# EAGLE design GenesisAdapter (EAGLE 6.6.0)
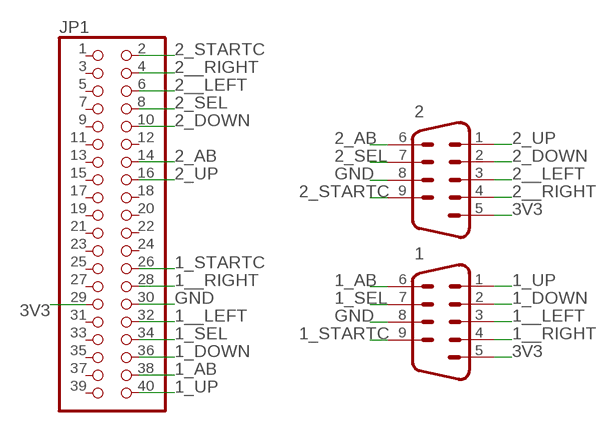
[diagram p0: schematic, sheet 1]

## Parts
1  M09H  [M09H]
2  M09H  [M09H]
JP1  PINHD-2X20  [2X20]

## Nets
1__LEFT: 1.3 JP1.32
1__RIGHT: 1.4 JP1.28
1_AB: 1.6 JP1.38
1_DOWN: 1.2 JP1.36
1_SEL: 1.7 JP1.34
1_STARTC: 1.9 JP1.26
1_UP: 1.1 JP1.40
2__LEFT: 2.3 JP1.6
2__RIGHT: 2.4 JP1.4
2_AB: 2.6 JP1.14
2_DOWN: 2.2 JP1.10
2_SEL: 2.7 JP1.8
2_STARTC: 2.9 JP1.2
2_UP: 2.1 JP1.16
3V3: 1.5 2.5 JP1.29
GND: 1.8 2.8 JP1.30
Unconnected: JP1.1 JP1.3 JP1.5 JP1.7 JP1.9 JP1.11 JP1.12 JP1.13 JP1.15 JP1.17 JP1.18 JP1.19 JP1.20 JP1.21 JP1.22 JP1.23 JP1.24 JP1.25 JP1.27 JP1.31 JP1.33 JP1.35 JP1.37 JP1.39

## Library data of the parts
1 2 = con-subd:M09: SUB-D; OC_FARNELL: unknown; OC_NEWARK: unknown
JP1 = pinhead:PINHD-2X20: PIN HEADER

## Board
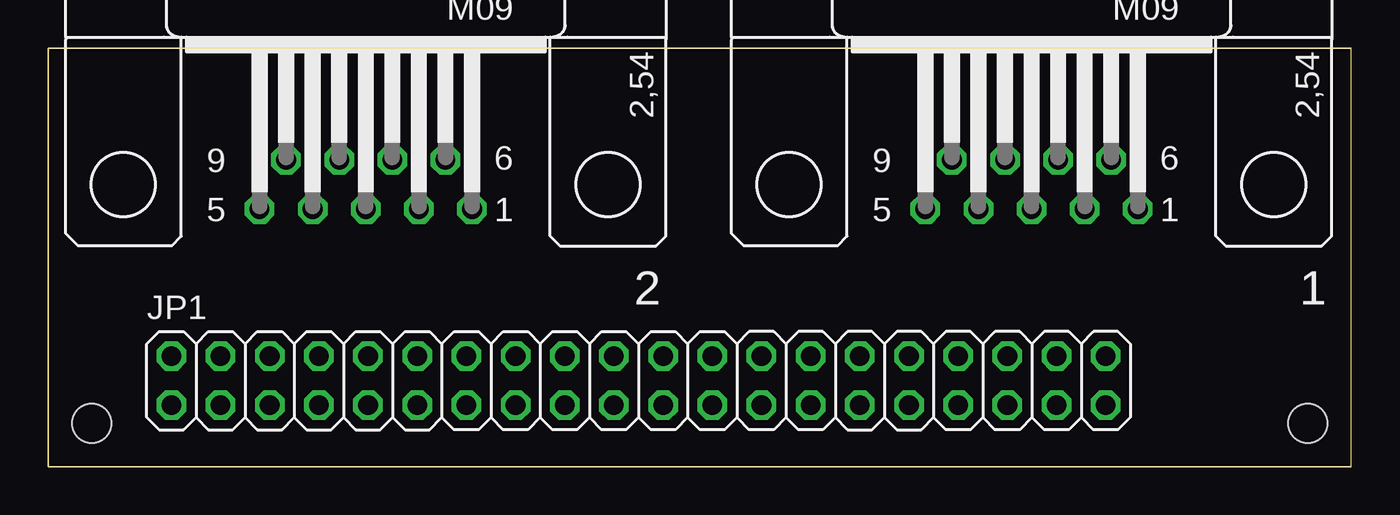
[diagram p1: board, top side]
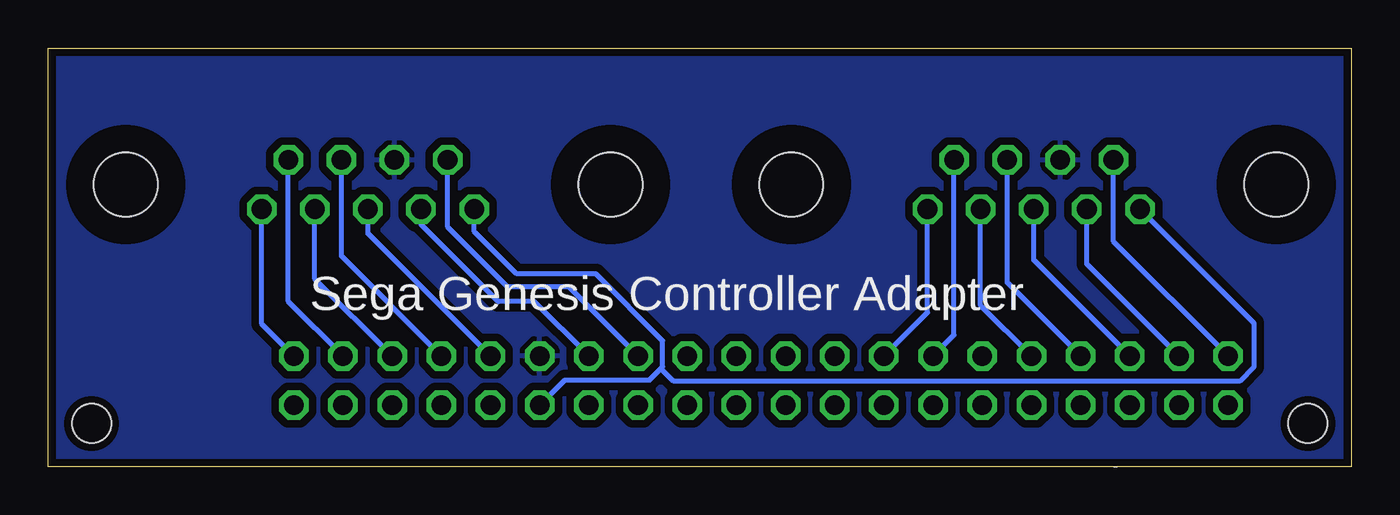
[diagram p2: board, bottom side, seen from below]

Size 67.28 x 21.62 mm. Coordinates in mm from the lower left corner, seen from the top.
Outline: 0,0 67.28,0 67.28,21.61 0,21.61 0,0
Copper layers (1*16): Top 0.0356mm / dielectric 1.5011mm / Bottom 0.0356mm
Design rules "LaenPCBOrder": minimum track width 6mil, minimum drill 13mil, track to track 6mil, track to pad 6mil, pad to pad 6mil, via to via 6mil, smd to smd 6mil, copper to edge 15mil, drill to drill 6mil, minimum pad ring 7mil, minimum via ring 7mil, stop-mask expansion 3mil, vias tented up to drill 0mil, thermal gap 10mil
Holes 2 mm at 2.24,2.24 65.05,2.24

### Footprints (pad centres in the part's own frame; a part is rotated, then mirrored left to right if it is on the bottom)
M09H = drill 1.016 octagon: 1 -5.486,1.27; 2 -2.743,1.27; 3 0,1.27; 4 2.743,1.27; 5 5.486,1.27; 6 -4.115,-1.27; 7 -1.372,-1.27; 8 1.372,-1.27; 9 4.115,-1.27 | hole 3.302: 12.522,0; -12.522,0
2X20 = drill 1.016 octagon: 1 -24.13,-1.27; 2 -24.13,1.27; 3 -21.59,-1.27; 4 -21.59,1.27; 5 -19.05,-1.27; 6 -19.05,1.27; 7 -16.51,-1.27; 8 -16.51,1.27; 9 -13.97,-1.27; 10 -13.97,1.27; 11 -11.43,-1.27; 12 -11.43,1.27; 13 -8.89,-1.27; 14 -8.89,1.27; 15 -6.35,-1.27; 16 -6.35,1.27; 17 -3.81,-1.27; 18 -3.81,1.27; 19 -1.27,-1.27; 20 -1.27,1.27; 21 1.27,-1.27; 22 1.27,1.27; 23 3.81,-1.27; 24 3.81,1.27; 25 6.35,-1.27; 26 6.35,1.27; 27 8.89,-1.27; 28 8.89,1.27; 29 11.43,-1.27; 30 11.43,1.27; 31 13.97,-1.27; 32 13.97,1.27; 33 16.51,-1.27; 34 16.51,1.27; 35 19.05,-1.27; 36 19.05,1.27; 37 21.59,-1.27; 38 21.59,1.27; 39 24.13,-1.27; 40 24.13,1.27

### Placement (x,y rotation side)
1  50.78,14.58 180 top
2  16.39,14.58 180 top
JP1  30.48,4.45 0 top

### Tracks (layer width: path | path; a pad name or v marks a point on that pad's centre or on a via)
1__LEFT
  Bottom 0.254: JP1.32 50.78,12.04 1.3
1__RIGHT
  Bottom 0.254: JP1.28 42.19,8.53 44.06,8.53 48.04,12.51 1.4
1_AB
  Bottom 0.254: JP1.38 54.89,8.54 1.6
1_DOWN
  Bottom 0.254: JP1.36 53.52,9.71 1.2
1_SEL
  Bottom 0.254: JP1.34 52.15,10.88 1.7
1_STARTC
  Bottom 0.254: JP1.26 40.4,9.28 43.56,9.28 46.66,12.38 1.9
1_UP
  Bottom 0.254: JP1.40 56.27,7.37 1.1
2__LEFT
  Bottom 0.254: JP1.6 16.39,10.68 2.3
2__RIGHT
  Bottom 0.254: JP1.4 13.65,10.47 2.4
2_AB
  Bottom 0.254: JP1.14 20.51,6.8 2.6
2_DOWN
  Bottom 0.254: JP1.10 19.14,8.34 2.2
2_SEL
  Bottom 0.254: JP1.8 17.77,9.51 2.7
2_STARTC
  Bottom 0.254: JP1.2 12.28,11.64 2.9
2_UP
  Bottom 0.254: JP1.16 21.88,7.96 2.1
3V3
  Bottom 0.254: JP1.29 40.6,4.48 36.24,4.48 35.68,5.03 | 35.68,5.03 35.56,5.16 35.56,6.51 39.01,9.96 43.1,9.96 45.29,12.15 1.5 | 2.5 5.01,7.42 5.01,5.16 5.76,4.41 34.99,4.41 35.61,5.03 35.68,5.03
GND
  pour Bottom (isolate 0.406): 0,21.55 67.21,21.55 67.21,0.07 0.04,0.07 0.04,21.51 0,21.51

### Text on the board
tPlace: /home/stephen/Pictures/dolphin.bmp
bPlace: Sega Genesis Controller Adapter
